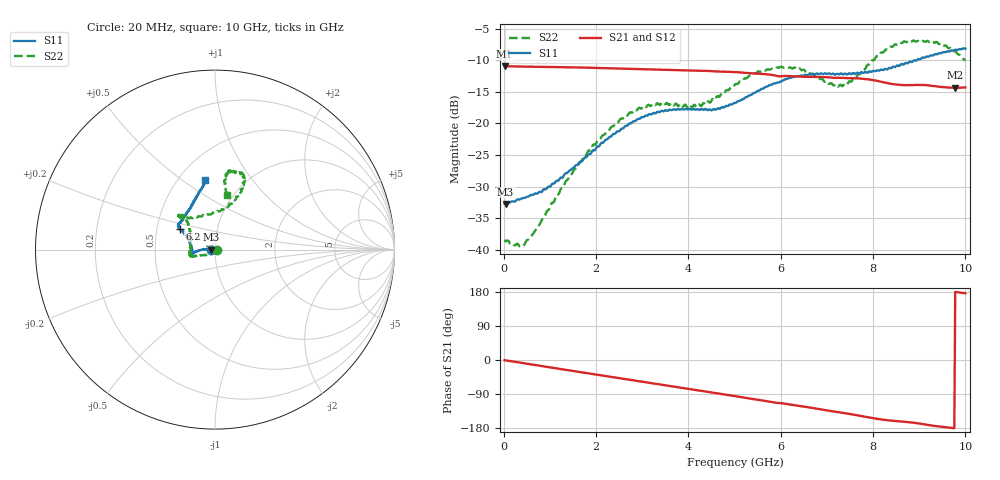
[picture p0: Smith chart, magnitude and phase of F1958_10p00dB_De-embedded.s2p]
! Integrated Device Technology
! Corporate Headquarters
! 6024 Silver Creek Valley Road
! San Jose, CA 95138  USA
! Phone:  1-408-284-8200
! Toll Free:  1-800-223-1366
! Webpage:  http://www.idt.com/
! Timing and RF Division
! 515 Groton Road, Suite 102
! Westford, MA 01886-6024
! Device:  F1958
! Description: 7-bit 0.25 dB Digital Step Attenuator
! Frequency:  0.001 -  6.000 GHz
! Package:  4x4 mm Thin QFN Plastic Package: 24 pin
! Ports:  2 RF, 12 DC
!  Pin  1  = D0
!  Pin  2  = VDD
!  Pin  3  = VMODE
!  Pin  4  = GND
!  Pin  5  = RF1  =  Port 1
!  Pin  6  = GND
!  Pin  7  = GND
!  Pin  8  = GND
!  Pin  9  = GND
!  Pin 10  = GND
!  Pin 11  = GND
!  Pin 12  = GND
!  Pin 13  = GND
!  Pin 14  = RF2  =  Port 2
!  Pin 15  = GND
!  Pin 16  = LE
!  Pin 17  = CLK
!  Pin 18  = DATA
!  Pin 19  = D6
!  Pin 20  = D5
!  Pin 21  = D4
!  Pin 22  = D3
!  Pin 23  = D2
!  Pin 24  = D1
! State:  40
! Atten State:  10.00 dB
! Voltage:  +3.30 Volts
! Current:  0.258 mA
! Data:  The device was measured on a F1958 evaluation board which has
!  individual transmission lines to the RF pins.  Data was collected
!  using a calibrated network analyzer.  The evaluation board was
!  de-embedded using Automatic Fixture Removal (AFR).
!  The reference plane is the edge of the package pin.
! Misc:
!  Action Tracker AT0419
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# GHz S dB R 50
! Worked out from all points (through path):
!   500 points, 20 MHz to 10 GHz, reference 50 ohm
!   highest |S21| = -10.94 dB at 20 MHz (marker M1); lowest = -14.4 dB at 9.78 GHz (marker M2)
!   group delay of S21, straight-line fit = 51.9 ps
!   lowest |S11| = -32.8 dB at 40 MHz (marker M3), VSWR 1.05, Z = 47.7 - j0.0753 ohm
!   |S11| at or under -10 dB: start of sweep to 8.946 GHz
!   |S22| runs from -39.4 to -6.9 dB; largest |S21 - S12| = 0.00086
!   S11 on the Smith chart (normalised r, x): 20 MHz: 0.95, -0.00; 6.2 GHz: 0.65, +0.16; 10 GHz: 0.67, +0.61
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0.02  -32.72 -178.1  -10.94 -0.5  -10.94 -0.5  -38.43 -9.2
0.04  -32.75 -178.0  -10.95 -0.9  -10.94 -0.9  -38.68 -14.5
0.44  -31.81 175.3  -11.00 -8.6  -11.00 -8.6  -39.27 -57.8
0.96  -30.03 175.8  -11.04 -18.6  -11.04 -18.6  -33.73 -107.9
1.7  -25.97 178.6  -11.16 -32.6  -11.15 -32.6  -25.77 -147.1
2.58  -20.81 -175.5  -11.33 -49.4  -11.32 -49.4  -19.22 -161.5
2.92  -19.29 -173.1  -11.40 -55.8  -11.39 -55.9  -17.57 -164.1
3.36  -18.21 -170.7  -11.51 -64.1  -11.51 -64.2  -16.98 -166.0
4.24  -17.87 -175.0  -11.66 -80.7  -11.67 -80.7  -17.01 166.6
4.64  -17.60 176.3  -11.78 -88.2  -11.79 -88.3  -15.69 148.8
5.02  -16.76 165.1  -11.88 -95.6  -11.89 -95.6  -13.78 137.1
5.54  -14.78 154.2  -12.14 -105.6  -12.15 -105.6  -11.78 134.0
6.2  -12.78 149.5  -12.51 -117.4  -12.53 -117.4  -11.11 137.4
6.68  -12.20 146.5  -12.63 -126.2  -12.65 -126.2  -12.16 133.2
7.1  -12.21 142.1  -12.75 -135.0  -12.76 -134.9  -13.64 116.0
7.36  -12.24 139.4  -12.80 -139.8  -12.80 -139.7  -13.92 94.6
7.9  -11.85 128.8  -13.03 -151.3  -13.02 -151.3  -10.67 70.0
8.34  -11.25 119.4  -13.66 -159.4  -13.66 -159.5  -8.16 65.9
8.74  -10.50 112.0  -13.95 -163.7  -13.96 -163.7  -7.08 69.4
9.24  -9.25 103.1  -14.03 -172.5  -14.03 -172.6  -7.09 78.4
9.78  -8.34 98.6  -14.37 179.6  -14.39 179.7  -8.56 81.2
10  -8.16 98.0  -14.30 176.1  -14.33 176.1  -10.08 77.2
